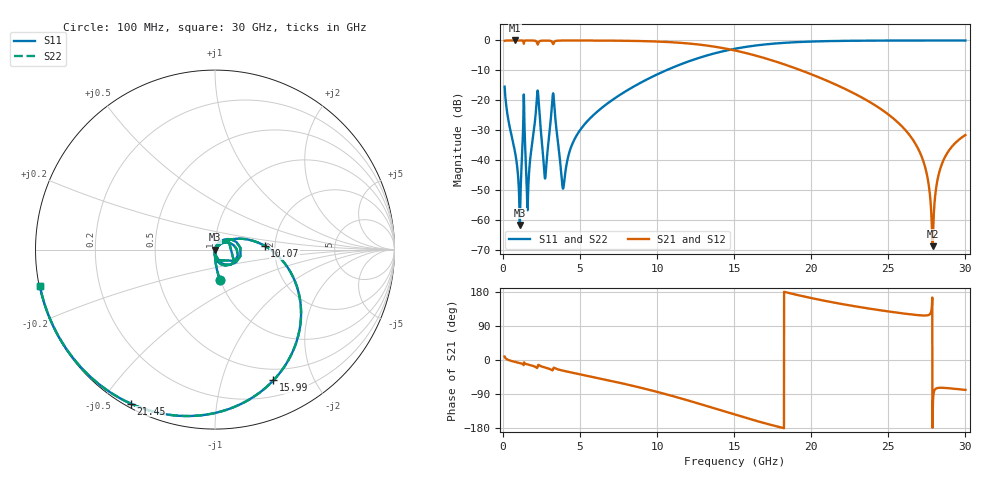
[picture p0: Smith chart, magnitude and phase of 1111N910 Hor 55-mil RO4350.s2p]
# GHz S MA R 50
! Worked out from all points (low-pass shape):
!   3201 points, 100 MHz to 30 GHz, reference 50 ohm
!   highest |S21| = -0.01 dB at 791.4 MHz (marker M1); lowest = -68.6 dB at 27.87 GHz (marker M2)
!   |S21| within 3 dB of the highest: start of sweep to 14.73 GHz
!   lowest |S11| = -61.5 dB at 1.09 GHz (marker M3), VSWR 1.00, Z = 50.1 - j0.00905 ohm
!   |S11| at or under -10 dB: start of sweep to 10.57 GHz
!   |S22| runs from -61.5 to 0.0 dB; largest |S21 - S12| = 0
!   S11 on the Smith chart (normalised r, x): 100 MHz: 1.00, -0.34; 10.07 GHz: 1.76, +0.08; 15.99 GHz: 0.37, -1.48; 21.45 GHz: 0.01, -0.59; 30 GHz: 0.00, -0.10
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0.1  0.1696 -80.9  0.9853 9.0  0.9853 9.0  0.1696 -80.9
0.7914375  0.01306 -92.7  0.9993 -5.1  0.9993 -5.1  0.01306 -92.7
1.090437  0.0008429 -6.2  0.999 -8.0  0.999 -8.0  0.0008429 -6.2
1.342719  0.1257 7.8  0.8808 -12.3  0.8808 -12.3  0.1257 7.8
1.548281  0.002899 -68.7  0.9983 -11.2  0.9983 -11.2  0.002899 -68.7
1.660406  0.00485 59.9  0.9983 -12.4  0.9983 -12.4  0.00485 59.9
2.221031  0.135 12.1  0.8832 -20.4  0.8832 -20.4  0.135 12.1
2.725594  0.004974 -15.0  0.9947 -19.9  0.9947 -19.9  0.004974 -15.0
3.286219  0.1125 -51.6  0.9016 -20.6  0.9016 -20.6  0.1125 -51.6
3.902906  0.003408 -13.8  0.9963 -28.3  0.9963 -28.3  0.003408 -13.8
5.089563  0.03451 48.1  0.9968 -38.5  0.9968 -38.5  0.03451 48.1
10.06978  0.2768 4.5  0.9569 -84.9  0.9569 -84.9  0.2768 4.5
15.05  0.7269 -54.5  0.6797 -144.2  0.6797 -144.2  0.7269 -54.5
15.99372  0.7976 -65.9  0.5954 -155.5  0.5954 -155.5  0.7976 -65.9
20.03956  0.9589 -107.3  0.2703 163.1  0.2703 163.1  0.9589 -107.3
21.45047  0.9782 -118.7  0.1905 151.7  0.1905 151.7  0.9782 -118.7
25.01978  0.9952 -142.6  0.05789 128.0  0.05789 128.0  0.9952 -142.6
27.08475  0.9969 -154.1  0.01294 117.8  0.01294 117.8  0.9969 -154.1
27.51456  0.9969 -156.4  0.00562 117.8  0.00562 117.8  0.9969 -156.4
27.86962  0.997 -158.2  0.000372 -157.6  0.000372 -157.6  0.997 -158.2
28.51434  0.9969 -161.4  0.009248 -73.3  0.009248 -73.3  0.9969 -161.4
30  0.9966 -168.4  0.02651 -78.9  0.02651 -78.9  0.9966 -168.4
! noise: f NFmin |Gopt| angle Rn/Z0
0.1  0.0006782  0.7388  1.191  0.0005197
3.417  0.03318  0.8127  24.86  0.03528
6.743  0.01678  0.4401  45.85  0.004329
10.06  0.02436  0.4503  63.13  0.005663
13.39  0.03618  0.5231  78.8  0.008468
16.7  0.05753  0.6435  95.66  0.01455
20.03  0.1047  0.7823  114.7  0.0298
23.35  0.2426  0.8999  134  0.08208
26.67  1.266  0.9797  152.1  0.8356
30  1.002  0.9736  168.3  0.0923
